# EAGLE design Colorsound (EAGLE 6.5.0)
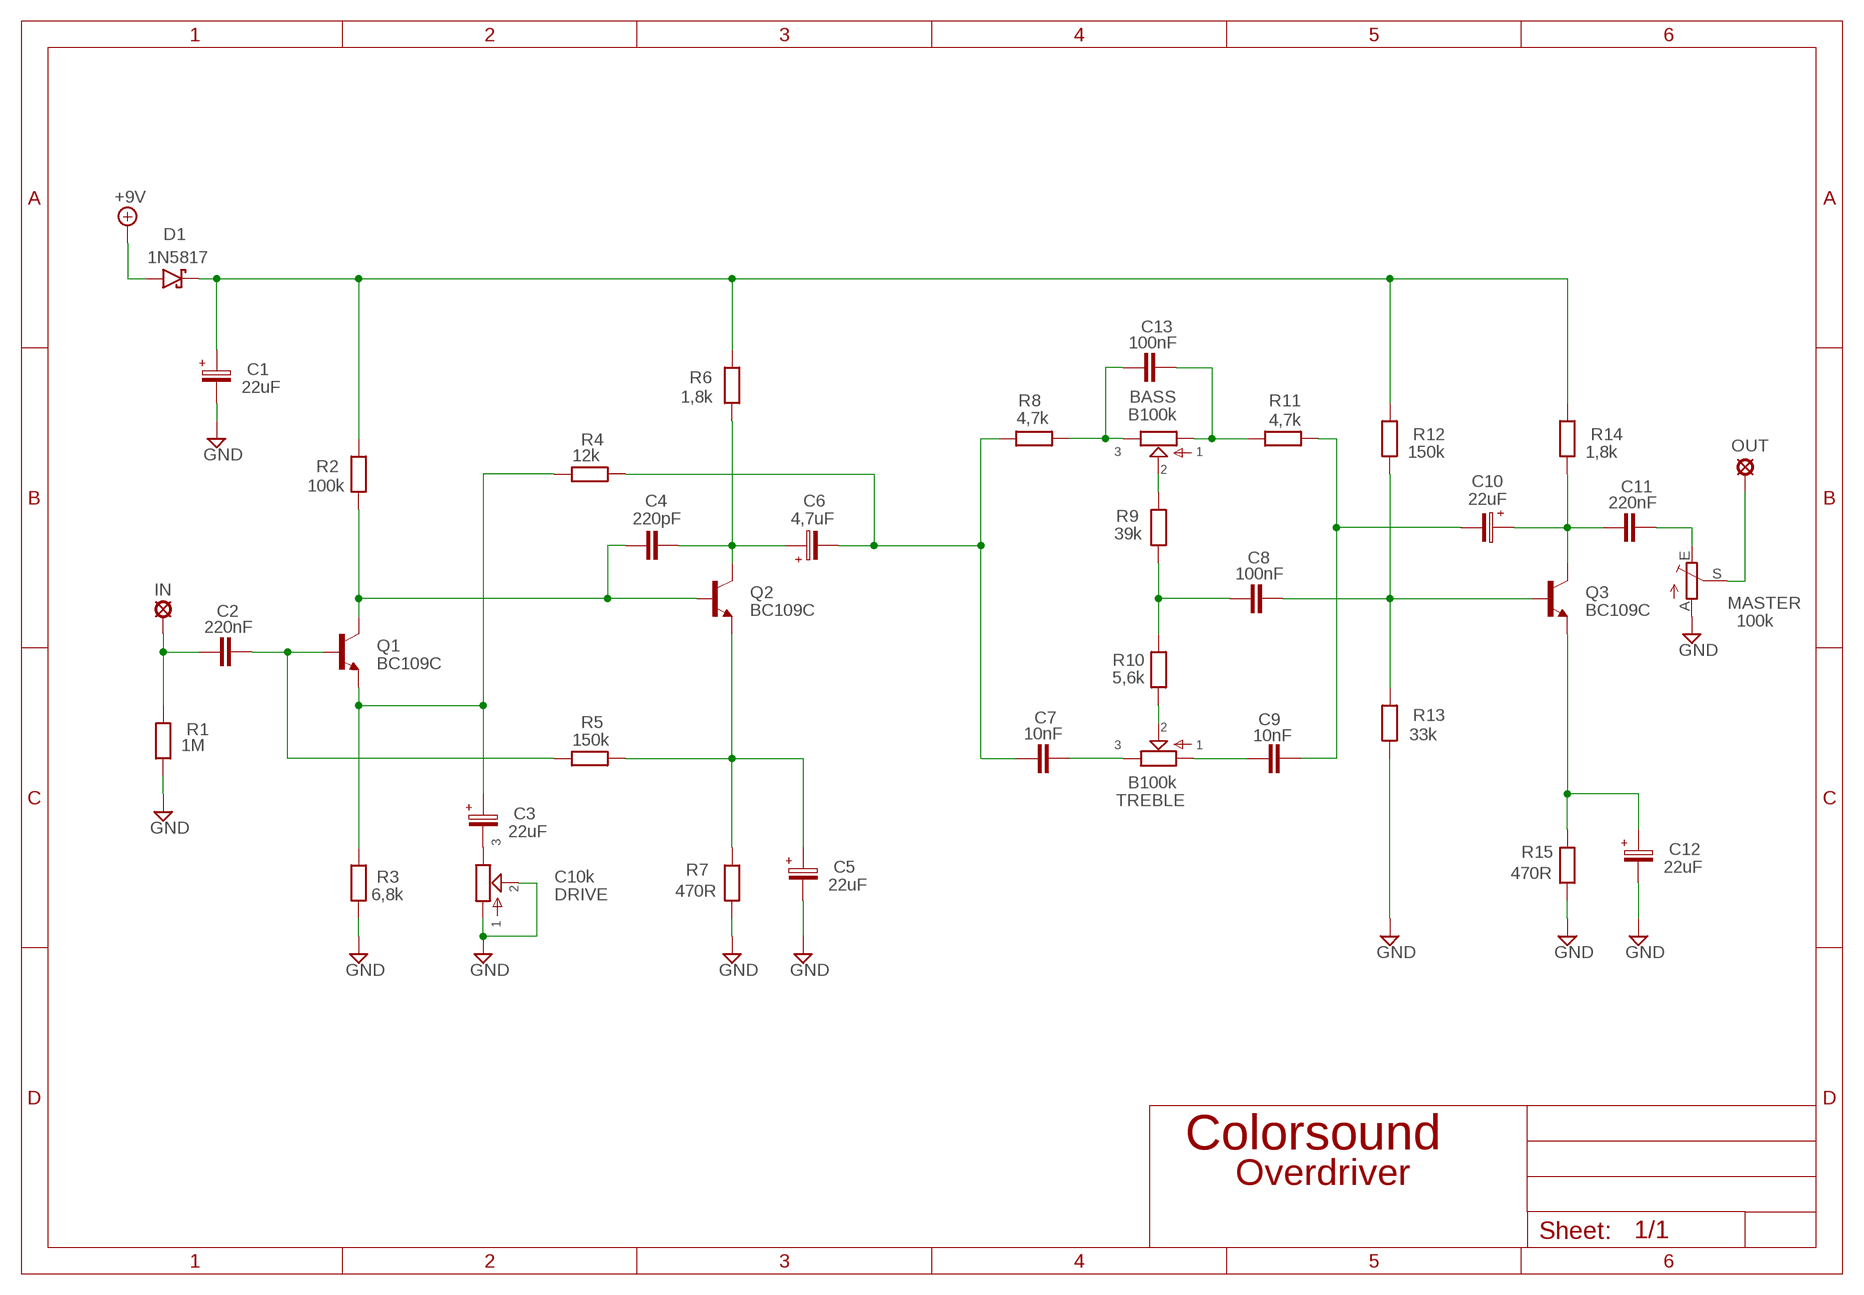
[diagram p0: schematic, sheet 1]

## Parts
+9V  +9V  +9V(T)1  [ROUND]
BASS  B100k  POT-EU16MM  [16MM]
C1  22uF  063-EU  [063_025]
C2  220nF  C10/4  [C10B4]
C3  22uF  063-EU  [063_025]
C4  220pF  050X030_0502  [050X030_050]
C5  22uF  063-EU  [063_025]
C6  4,7uF  050-EU  [050_020]
C7  10nF  C10/4  [C10B4]
C8  100nF  C10/4  [C10B4]
C9  10nF  C10/4  [C10B4]
C10  22uF  050-EU  [050_020]
C11  220nF  C10/4  [C10B4]
C12  22uF  063-EU  [063_025]
C13  100nF  C10/4  [C10B4]
D1  1N5817  [DO41-3]
DRIVE  C10k  POT-EU16MM  [16MM]
GND  GND  GND(T)1  [ROUND]
GND3  GND  GND(T)1  [ROUND]
IN  MCS10B  [MCS10B]
MASTER  100k  TRIM_EU-PT10  [PT-10]
OUT  MCS10B  [MCS10B]
Q1  BC109C  BC108C  [TO18]
Q2  BC109C  BC108C  [TO18]
Q3  BC109C  BC108C  [TO18]
R1  1M  6MM-EU3  [R0207/3]
R2  100k  6MM-EU3  [R0207/3]
R3  6,8k  6MM-EU3  [R0207/3]
R4  12k  6MM-EU3  [R0207/3]
R5  150k  6MM-EU3  [R0207/3]
R6  1,8k  6MM-EU3  [R0207/3]
R7  470R  6MM-EU3  [R0207/3]
R8  4,7k  6MM-EU3  [R0207/3]
R9  39k  6MM-EU3  [R0207/3]
R10  5,6k  6MM-EU3  [R0207/3]
R11  4,7k  6MM-EU3  [R0207/3]
R12  150k  6MM-EU3  [R0207/3]
R13  33k  6MM-EU3  [R0207/3]
R14  1,8k  6MM-EU3  [R0207/3]
R15  470R  6MM-EU3  [R0207/3]
TREBLE  B100k  POT-EU16MM  [16MM]

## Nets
+9V: +9V.1(+9V) D1.A
GND: C1.- C5.- C12.- DRIVE.1 DRIVE.2 GND3.1(GND) GND.1(GND) MASTER.A R1.1 R3.1 R7.1 R13.1 R15.1
N$1: C2.2 IN.MP R1.2
N$2: C2.1 Q1.2(B) R5.1
N$3: C3.+ Q1.1(E) R3.2 R4.1
N$4: C3.- DRIVE.3
N$5: C5.+ Q2.1(E) R5.2 R7.2
N$6: C4.1 Q1.3(C) Q2.2(B) R2.1
N$7: C1.+ D1.C R2.2 R6.2 R12.2 R14.2
N$8: C4.2 C6.+ Q2.3(C) R6.1
N$9: C8.2 Q3.2(B) R12.1 R13.2
N$10: C6.- C7.2 R4.2 R8.1
N$11: C12.+ Q3.1(E) R15.2
N$12: C10.+ C11.1 Q3.3(C) R14.1
N$13: R10.1 TREBLE.2
N$14: C7.1 TREBLE.3
N$15: C9.1 TREBLE.1
N$16: C8.1 R9.1 R10.2
N$17: C9.2 C10.- R11.2
N$18: BASS.2 R9.2
N$19: BASS.3 C13.1 R8.2
N$20: BASS.1 C13.2 R11.1
N$21: C11.2 MASTER.E
N$22: MASTER.S OUT.MP

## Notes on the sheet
- Overdriver

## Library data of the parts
+9V = gm-supply:+9V(T): +9V Voltage Supply
BASS DRIVE TREBLE = gm-pots:POT-EU
C1 C3 C5 C12 = Elektrolyytit:063-EU
C2 C7-C9 C11 C13 = capacitor-wima:C: CAPACITOR
C4 = Keraamiset kondensaattorit:050X030_050: 120 - 150pF
C6 C10 = Elektrolyytit:050-EU
D1 = Diodit:1N5817
GND GND3 = gm-supply:GND(T): Ground
IN OUT = Padit:MCS10B: SOLDER PAD
MASTER = pot:TRIM_EU-: POTENTIOMETER
Q1-Q3 = transistor-npn:BC108C: NPN Transistor
R1-R15 = Vastukset:6MM-EU: 6mm Resistors (European schematic symbol)

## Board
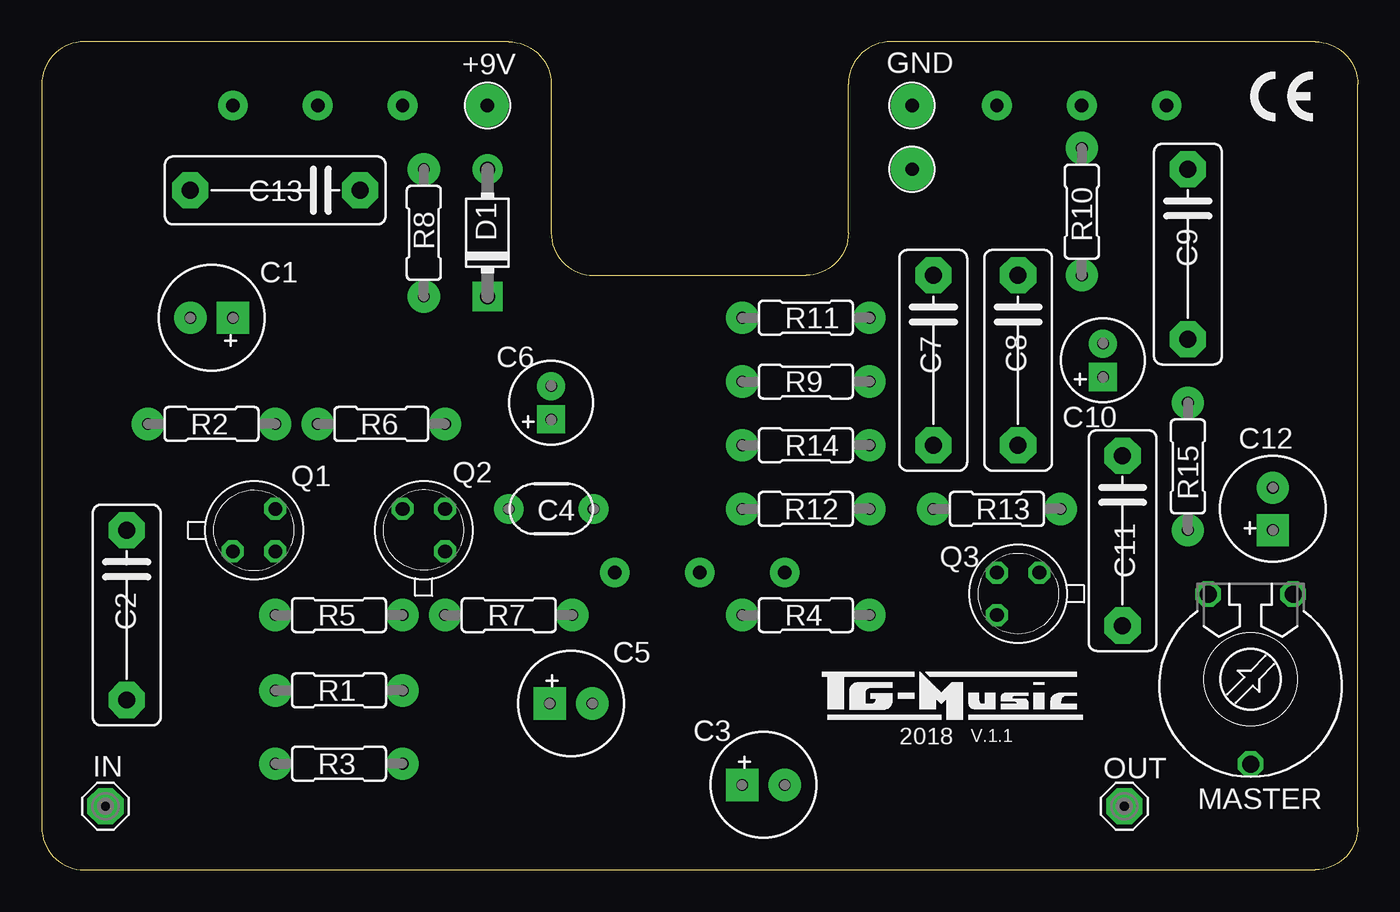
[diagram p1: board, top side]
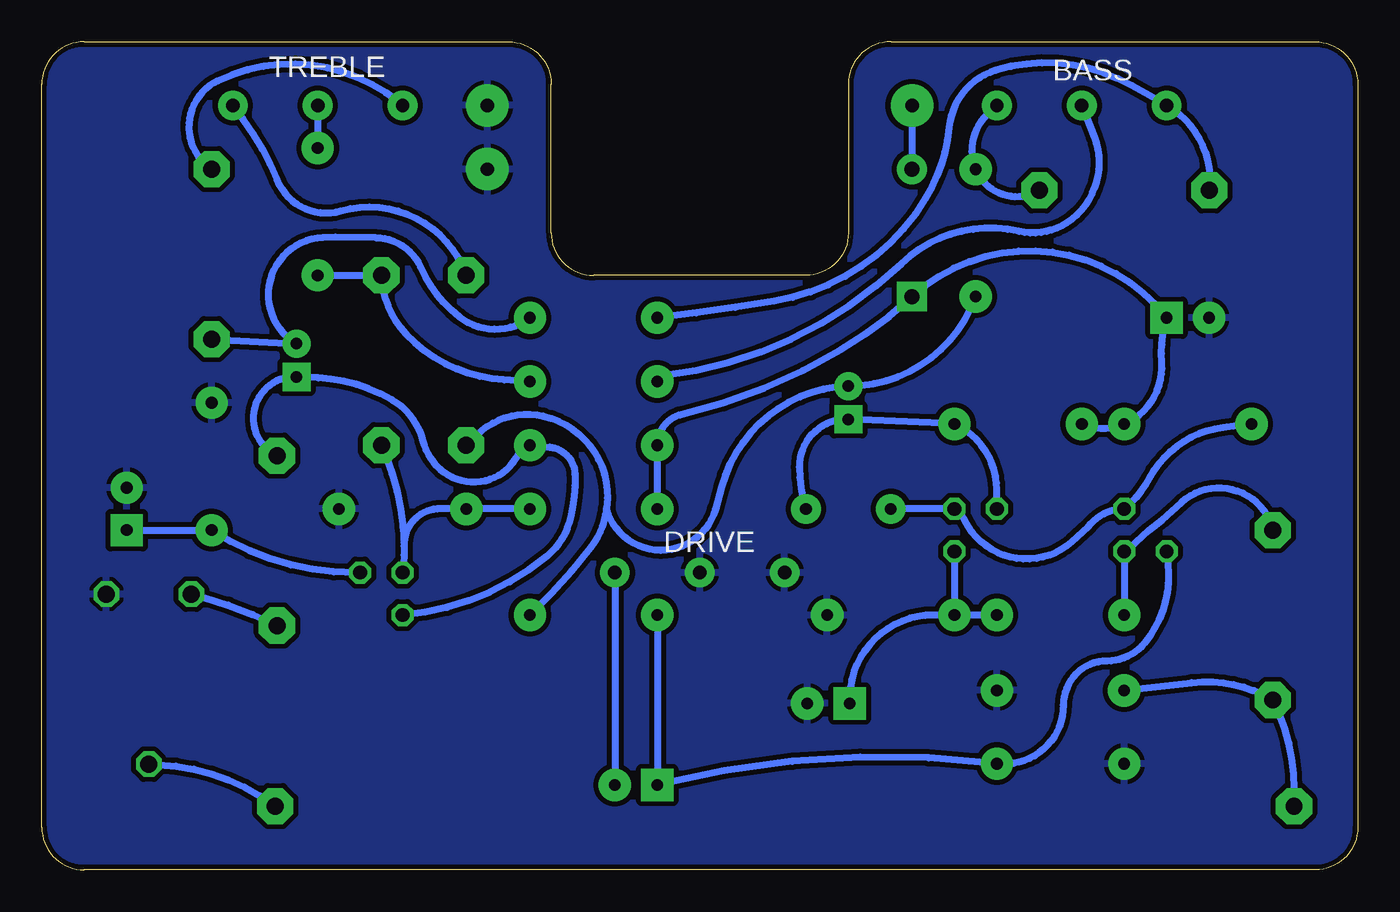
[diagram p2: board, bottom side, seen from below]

Size 78.74 x 49.53 mm. Coordinates in mm from the lower left corner, seen from the top.
Outline: 7.62,49.53 3.81,49.53
Outline: 78.74,2.54 78.74,46.99 arc90 76.2,49.53 50.8,49.53 arc90 48.26,46.99 48.26,38.1 arc-90 45.72,35.56 33.02,35.56 arc-90 30.48,38.1 30.48,46.99 arc90 27.94,49.53 2.54,49.53 arc90 0,46.99 0,2.54 arc90 2.54,0 76.2,0 arc90 78.74,2.54
Copper layers (1*16): Top 0.035mm / dielectric 1.5mm / Bottom 0.035mm
Design rules "ITEADstudio": minimum track width 10mil, minimum drill 12mil, track to track 12mil, track to pad 12mil, pad to pad 12mil, via to via 12mil, smd to smd 0mil, copper to edge 12mil, drill to drill 12mil, minimum pad ring 10mil, minimum via ring 6mil, stop-mask expansion 4mil, vias tented up to drill 100mil, thermal gap 10mil

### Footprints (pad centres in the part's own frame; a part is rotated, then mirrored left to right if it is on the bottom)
ROUND = drill 0.8 pad 2.54: 1 0,0
16MM = drill 0.8 pad 1.778: 1 5.08,0; 2 0,0; 3 -5.08,0
063_025 = drill 0.7 pad 1.93 square: + -1.27,0 | drill 0.7 pad 1.93: - 1.27,0
C10B4 = drill 1.016 pad 2.159 octagon: 1 -5.08,0; 2 5.08,0
050X030_050 = drill 0.7 pad 1.778: 1 -2.54,0; 2 2.54,0
050_020 = drill 0.7 pad 1.676 square: + -1,0 | drill 0.7 pad 1.676: - 1,0
DO41-3 = drill 0.9 pad 1.778: A 3.81,0 | drill 0.9 pad 1.778 square: C -3.81,0
MCS10B = drill 1.016 pad 2.159 octagon: MP 0,0
PT-10 = drill 1.016 octagon: A -2.54,-5.08; E 2.54,-5.08; S 0,5.08
TO18 = drill 0.813 octagon: 1 -1.27,-1.27; 2 1.27,-1.27; 3 1.27,1.27
R0207/3 = drill 0.7 pad 1.93: 1 -3.81,0; 2 3.81,0

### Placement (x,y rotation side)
+9V  26.67,45.72 0 top
BASS  16.51,45.72 0 bottom
C1  10.16,33.02 180 top
C2  5.08,15.24 270 top
C3  43.18,5.08 0 top
C4  30.48,21.59 0 top
C5  31.66,9.95 0 top
C6  30.48,27.94 90 top
C7  53.34,30.48 270 top
C8  58.42,30.48 270 top
C9  68.58,36.83 270 top
C10  63.5,30.48 90 top
C11  64.67,19.69 270 top
C12  73.66,21.59 90 top
C13  13.97,40.64 180 top
D1  26.67,38.1 90 top
DRIVE  39.37,17.78 0 bottom
GND  52.07,45.72 0 top
GND3  52.07,41.91 0 top
IN  3.81,3.81 0 top
MASTER  72.33,11.41 180 top
OUT  64.77,3.81 0 top
Q1  12.7,20.32 0 top
Q2  22.86,20.32 90 top
Q3  58.42,16.51 180 top
R1  17.78,10.74 180 top
R2  10.16,26.67 0 top
R3  17.78,6.35 0 top
R4  45.72,15.24 0 top
R5  17.78,15.24 0 top
R6  20.32,26.67 180 top
R7  27.94,15.24 180 top
R8  22.86,38.1 90 top
R9  45.72,29.21 180 top
R10  62.23,39.37 270 top
R11  45.72,33.02 0 top
R12  45.72,21.59 180 top
R13  57.15,21.59 180 top
R14  45.72,25.4 180 top
R15  68.58,24.13 270 top
TREBLE  62.23,45.72 0 bottom

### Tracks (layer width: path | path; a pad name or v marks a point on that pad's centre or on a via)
+9V
  Bottom 0.406: +9V.1 D1.A
GND
  pour Bottom: 0,2.54 0,46.99 arc-90 2.54,49.53 27.94,49.53 arc-90 30.48,46.99 30.48,38.1 arc90 33.02,35.56 45.72,35.56 arc90 48.26,38.1 48.26,46.99 arc-90 50.8,49.53 76.2,49.53 arc-90 78.74,46.99 78.74,2.54 arc-90 76.2,0 2.54,0 arc-90
N$1
  Bottom 0.406: R1.2 9.93,11.2 arc37 C2.2 arc27 3.81,4.84 IN.MP
N$2
  Bottom 0.406: Q1.2 13.97,18.89 | 13.97,18.89 R5.1 | 13.97,18.89 arc10 11.69,20.95 10.53,21.99 arc118 C2.1
N$3
  Bottom 0.406: Q1.1 11.35,18.29 arc45 12.76,13.57 arc51 15,12.49 arc-90 17.61,9.87 arc97 R3.2 arc-21 C3.+ R4.1
N$4
  Bottom 0.406: DRIVE.3 C3.-
N$5
  Bottom 0.406: R5.2 R7.2 | Q2.1 R7.2 | R7.2 25.4,15.24 arc-93 C5.+
N$6
  Bottom 0.406: C4.1 Q2.2 arc31 23.49,20.88 arc-106 17.1,19.63 16.14,20.49 arc54 Q1.3 arc-21 12.46,23.45 arc54 8.07,26.45 R2.1
N$7
  Bottom 0.406: R12.2 R14.2 arc77 40.45,27.24 arc-17 30.95,31.09 arc-12 D1.C arc95 C1.+ arc-20 11.72,30.35 arc71 R2.2 arc47 R6.2
N$8
  Bottom 0.406: C4.2 arc16 33.41,24.09 arc93 C6.+ R6.1 arc65 21.59,22.74 Q2.3
N$9
  Bottom 0.406: R12.1 R13.2 54.88,21.6 arc-92 57.07,19.38 | 57.07,19.38 arc9 Q3.2 | C8.2 58.15,24.72 arc21 57.07,19.38
N$10
  Bottom 0.406: C7.2 52.69,26.03 arc57 48.72,27.14 arc78 44.9,22.23 44.96,21.62 | 44.96,21.62 arc32 45.9,19.28 arc8 R4.2 | 44.96,21.62 arc-149 38.44,21.57 38.06,22.91 arc72 30.51,28.94 C6.- arc-70 R8.1
N$11
  Bottom 0.406: Q3.1 59.97,17.78 arc33 R15.2 C12.+
N$12
  Bottom 0.406: Q3.3 arc-35 48.52,18.77 arc-38 47.09,21.08 arc-14 46.84,23.65 arc-83 48.35,25.28 R14.1 50.01,25.4 arc106 54.43,23.63 arc45 55.94,25.66 arc-45 57.79,28.12 arc-28 62.2,29.42 C10.+ arc-157 C11.1
N$13
  Bottom 0.406: TREBLE.2 R10.1
N$14
  Bottom 0.406: TREBLE.3 66.68,44.86 arc14 64.66,41.27 arc-84 60.84,39.41 arc86 C7.1
N$15
  Bottom 0.406: TREBLE.1 57.38,45.91 arc-65 68.21,47.2 arc-121 C9.1
N$16
  Bottom 0.406: R10.2 C8.1 arc-41 56.94,32.04 arc-43 51.06,29.3 R9.1
N$17
  Bottom 0.406: R11.2 arc74 53.76,33.09 arc28 56.08,36.06 arc-65 58.77,37.82 61.17,37.84 61.92,37.81 arc-148 C10.- C9.2
N$18
  Bottom 0.406: BASS.2 15.77,43.82 arc78 17.41,38.7 arc46 20.26,38.19 arc-56 27.32,36.25 arc37 41.57,29.55 R9.2
N$19
  Bottom 0.406: BASS.3 22.16,45.19 arc-70 R8.2 arc-98 C13.1
N$20
  Bottom 0.406: R11.1 arc-2 34.93,34.01 arc-50 25.85,40.17 arc-26 24.45,44.41 arc68 21.65,47.83 arc46 13.51,46.9 BASS.1 arc68 C13.2
N$21
  Bottom 0.406: MASTER.E 69.09,16.3 arc12 C11.2
N$22
  Bottom 0.406: MASTER.S 71.78,6.3 arc34 OUT.MP

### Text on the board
tNames: V.1.1 | 2018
